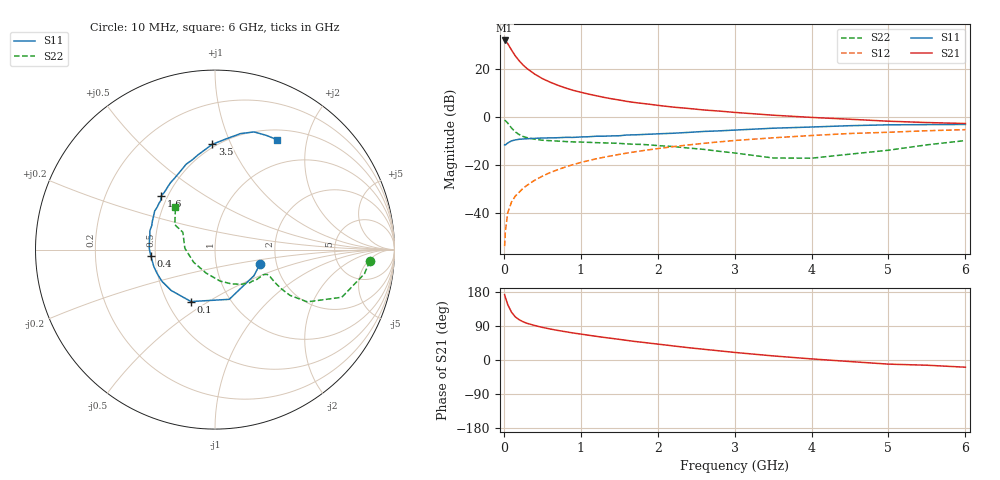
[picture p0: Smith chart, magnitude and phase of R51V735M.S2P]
! SIEMENS Small Signal Semiconductors
! BFR183
! Si NPN RF Bipolar Junction Transistor in SOT23
! VCE = 1.75 V  IC = 35 mA
! Common Emitter S-Parameters:  May  1996
# GHz  S  MA  R  50
!  f  S11  S21  S12  S22
! GHz  MAG  ANG  MAG  ANG  MAG  ANG  MAG  ANG
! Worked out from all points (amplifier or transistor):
!   36 points, 10 MHz to 6 GHz, reference 50 ohm
!   highest |S21| = 32.1 dB at 10 MHz (marker M1)
!   |S21| within 3 dB of that: start of sweep to 81.43 MHz
!   unconditionally stable (mu >= 1): start of sweep to 16.24 MHz; 263.4 MHz to 2.727 GHz
!   at 250 MHz: K = 0.99, MSG = 25.8 dB, |S12| = -29.8 dB
!   at 1.4 GHz: K = 1.10, MAG = 10.0 dB, |S12| = -16.2 dB
!   at 6 GHz: K = 0.96, MSG = 1.3 dB, |S12| = -5.2 dB
!   S11 on the Smith chart (normalised r, x): 10 MHz: 1.64, -0.28; 100 MHz: 0.66, -0.42; 400 MHz: 0.47, -0.04; 1.6 GHz: 0.46, +0.34; 3.5 GHz: 0.48, +0.85; 6 GHz: 0.63, +1.52
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0.01  0.2631 -17.8  40.17 172.5  0.002 81.6  0.8645 -4.3
0.02  0.2614 -33.7  39.34 165.1  0.0041 78.2  0.8434 -9.2
0.05  0.2882 -74.0  34.55 146.5  0.0099 72.5  0.7547 -20.6
0.1  0.3189 -114.8  25.35 126.0  0.0168 68.8  0.5912 -29.5
0.15  0.3341 -137.1  19.01 113.6  0.0224 68.9  0.4897 -31.4
0.2  0.3444 -149.1  15.04 106.2  0.0269 69.6  0.4312 -30.6
0.25  0.3492 -157.8  12.32 100.9  0.0325 70.5  0.3946 -29.4
0.3  0.3536 -164.5  10.42 96.9  0.0373 72.3  0.373 -28.3
0.4  0.3592 -174.2  7.96 91.1  0.0478 73.1  0.3452 -26.4
0.5  0.3663 179.1  6.415 86.1  0.0581 73.6  0.3289 -25.5
0.6  0.3681 173.4  5.4 81.9  0.0691 73.4  0.3217 -25.5
0.7  0.3709 168.3  4.655 78.1  0.0796 73.3  0.3156 -26.0
0.9  0.3769 159.3  3.643 71.3  0.1017 71.7  0.3036 -27.5
1.1  0.3888 152.0  3.038 65.4  0.1232 70.2  0.297 -30.5
1.3  0.3995 143.9  2.595 59.7  0.1448 68.1  0.2894 -33.4
1.6  0.4235 134.9  2.135 51.7  0.1771 64.6  0.2754 -39.1
2.2  0.4603 118.5  1.622 37.2  0.2413 57.2  0.2426 -52.9
3  0.536 100.2  1.256 20.0  0.3245 46.1  0.1781 -80.7
3.5  0.5867 91.5  1.098 10.8  0.3696 38.8  0.1399 -110.7
4.5  0.6624 77.5  0.903 -4.1  0.4547 25.0  0.1682 177.4
5.5  0.6976 65.8  0.771 -13.8  0.5194 12.7  0.2633 148.2
6  0.7035 60.6  0.736 -19.0  0.5472 5.0  0.3236 132.9
